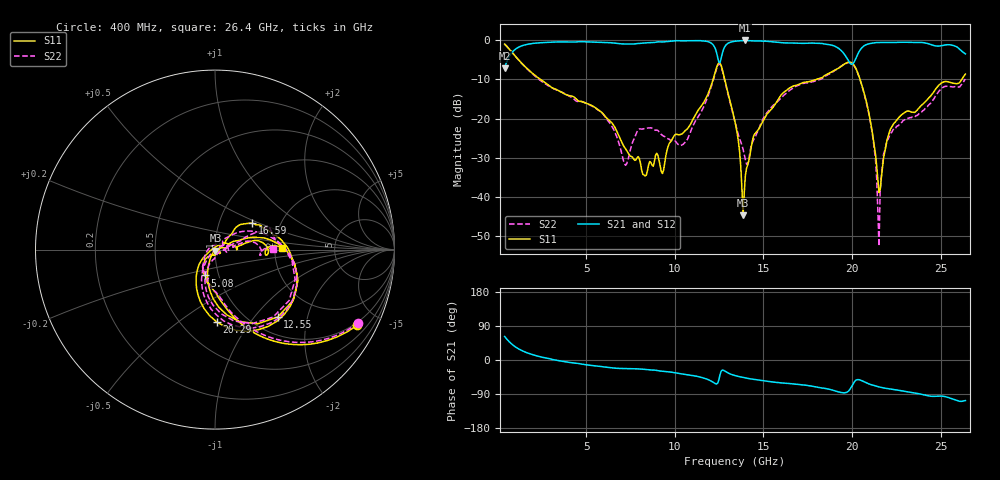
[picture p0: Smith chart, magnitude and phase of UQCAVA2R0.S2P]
!  Part Number  UQCAVA2R0
!  Description: RF capacitor  Mounting Orientation: Horizontal
!  Application:
# GHZ S DB R 50
! Freq  |S11|  S11 Ph  |S21|  S21 Ph  |S12|  S12 Ph  |S22|  S22 Ph
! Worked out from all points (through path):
!   401 points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, 400 MHz to 26.4 GHz, reference 50 ohm
!   highest |S21| = -0.01 dB at 13.98 GHz (marker M1); lowest = -7.2 dB at 400 MHz (marker M2)
!   group delay of S21, straight-line fit = 12.7 ps
!   lowest |S11| = -44.8 dB at 13.86 GHz (marker M3), VSWR 1.01, Z = 50.3 - j0.509 ohm
!   |S11| at or under -10 dB: 2.424 GHz to 12.16 GHz (9.74 GHz wide, 134 % of centre); 12.82 GHz to 17.99 GHz (5.166 GHz wide, 33.5 % of centre); 20.46 GHz to 26.19 GHz (5.738 GHz wide, 24.6 % of centre)
!   |S22| runs from -52.7 to -1.0 dB; largest |S21 - S12| = 0.0069
!   S11 on the Smith chart (normalised r, x): 400 MHz: 0.88, -3.82; 5.08 GHz: 0.86, -0.25; 12.55 GHz: 1.31, -1.33; 16.59 GHz: 1.44, +0.45; 20.29 GHz: 0.73, -0.71; 26.4 GHz: 2.18, +0.05
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0.4  -0.94 -28.0  -7.18 62.1  -7.21 62.2  -0.96 -27.2
1.765  -7.59 -72.4  -0.93 17.4  -0.95 17.4  -7.70 -71.2
4.755  -15.65 -107.0  -0.32 -10.9  -0.33 -10.8  -15.66 -105.0
5.08  -16.21 -111.5  -0.36 -13.1  -0.37 -12.9  -16.23 -109.8
7.225  -27.81 -123.3  -0.92 -22.6  -0.91 -22.4  -31.97 117.8
7.94  -29.75 -92.2  -0.79 -23.6  -0.78 -23.4  -22.89 13.8
9.11  -30.65 -42.7  -0.36 -28.6  -0.34 -28.4  -23.36 -11.6
10.54  -23.33 13.4  -0.10 -37.5  -0.09 -37.5  -26.30 32.7
12.1  -10.93 13.1  -0.83 -56.8  -0.82 -56.7  -11.30 20.1
12.555  -5.80 -47.0  -5.70 -38.9  -5.69 -38.9  -6.09 -49.3
13.4  -20.88 -112.9  -0.21 -41.1  -0.19 -41.1  -20.91 -111.4
13.855  -44.77 -61.3  -0.04 -46.0  -0.01 -46.0  -27.81 -85.2
13.985  -34.60 12.7  -0.01 -47.4  -0.01 -47.4  -30.51 -71.1
14.505  -23.97 34.9  -0.12 -51.3  -0.09 -51.3  -25.08 1.4
16.585  -11.89 35.1  -0.66 -62.7  -0.63 -62.8  -12.45 22.8
17.755  -10.31 22.3  -0.68 -69.2  -0.65 -69.3  -10.59 21.9
19.575  -6.05 -23.8  -3.57 -86.6  -3.54 -86.8  -6.06 -24.0
20.29  -7.87 -88.5  -3.89 -51.9  -3.86 -52.2  -7.97 -83.2
21.07  -21.49 -144.1  -0.75 -64.9  -0.72 -65.2  -21.70 -127.5
21.525  -38.93 142.2  -0.55 -71.0  -0.52 -71.3  -52.67 -28.7
22.11  -23.50 31.9  -0.54 -76.3  -0.52 -76.5  -24.46 20.6
26.4  -8.61 1.6  -3.45 -107.0  -3.43 -107.4  -9.88 0.9
